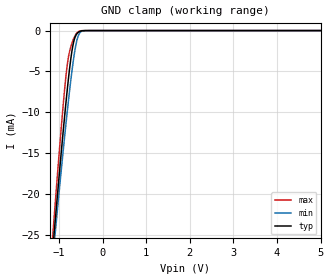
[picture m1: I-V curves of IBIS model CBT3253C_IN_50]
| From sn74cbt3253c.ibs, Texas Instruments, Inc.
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[Model]   CBT3253C_IN_50
Model_type  Input
Vinl=0.8
Vinh=2.0
| variable   typ   min   max
C_comp   2.57pF   1.85pF   3.37pF
[Temperature Range]   40   100   -40
| Ambient temperature   25   85   -40
[Voltage range]   5   4.5   5.5
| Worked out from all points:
|   GND clamp passes 1 mA (typ) near -0.64 V on its own axis
[GND Clamp]
| CBT3253C_IN_50
|   Voltage   I(typ)   I(min)   I(max)
-5V       -300.5mA   -278.7mA   -325.7mA
-1.16V    -27.92mA   -29.02mA   -26.33mA
-1.125V   -25.71mA   -27.01mA   -23.86mA
-1.09V    -23.52mA   -25.01mA   -21.42mA
-1.06V    -21.66mA   -23.31mA   -19.35mA
-910mV    -12.7mA    -15.06mA   -9.51mA
-815mV    -7.491mA   -10.15mA   -4.404mA
-760mV    -4.802mA   -7.489mA   -2.625mA
-680mV    -1.799mA   -4.025mA   -1.206mA
-605mV    -516.4uA   -1.559mA   -393.5uA
-545mV    -167.6uA   -476uA     -102.2uA
5V        123.2pA    298.9pA    65.41pA
